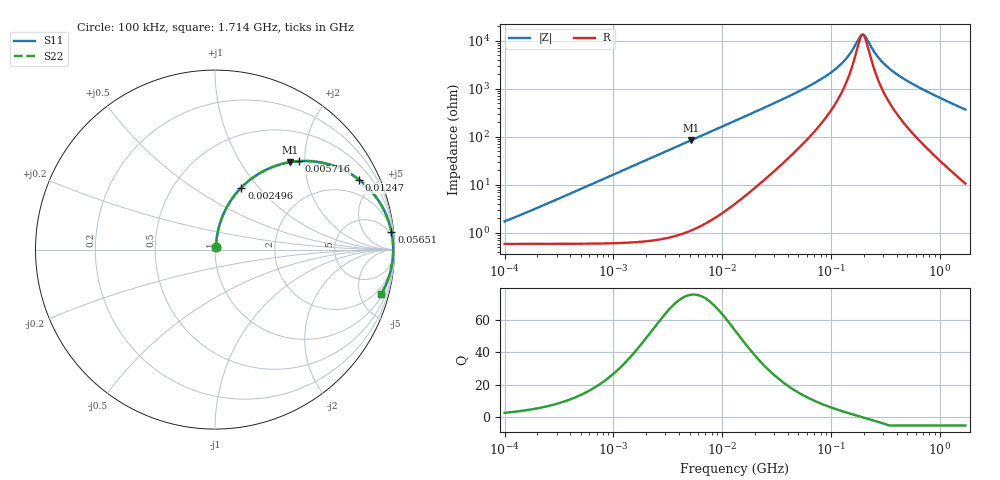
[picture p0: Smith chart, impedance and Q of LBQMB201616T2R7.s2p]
! LBQMB201616T2R7  S-PARAMETER MODEL  ( General Type )
! Model Generated by TAIYO YUDEN Corporation (http://www.ty-top.com)
! Version 1.0
! TAIYO YUDEN Control No. 191025NI43SB-FBB
! Copyright(c) 2019 TAIYO YUDEN CO.,LTD. All Rights Reserved.
! Product Description (link to TY-COMPAS)
! https://ds.yuden.co.jp/TYCOMPAS/or/detail?pn=LBQMB201616T2R7J&u=M
! Products Name : Inductors
! Characteristics :
!  Inductance : 2.7 uH , SRF(min) : 55 MHz , DC Resistance(max) : 0.767 Ohm , Rated Current : 310 mA
!  Case Size : 2.0 x 1.6 / 0.079 x 0.063 [mm/inch] , Thickness : 1.6 / 0.063 [mm/inch]
!  (Conditions: Temperature = 25 degC , DC Bias Current/Voltage = 0A / 0V)
! External Node Assignments :
!  1  o---GGG---o  2
! GND o---------o GND
! Frequency Range : 0.1MHz  -  1713.942084MHz  [ 402 STEP ]
# MHz S RI R 50
! Freq[MHz].  S11 Real  S11 Imag  S21 Real  S21 Imag  S12 Real  S12 Imag  S22 Real  S22 Imag
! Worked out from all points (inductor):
!   401 points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, 100 kHz to 1.714 GHz, reference 50 ohm
!   read as one part in series: L = 2.6 uH near 110.2 kHz
!   highest Q = 75.5 at 5.185 MHz (marker M1), where L = 2.61 uH
!   self-resonance near 191.1 MHz
!   S11 on the Smith chart (normalised r, x): 100 kHz: 1.01, +0.03; 2.496 MHz: 1.01, +0.82; 5.716 MHz: 1.02, +1.87; 12.47 MHz: 1.07, +4.09; 56.51 MHz: 3, +20; 1.714 GHz: 1.21, -7.37
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0.1  0.00613 0.0162  0.9939 -0.0162  0.9939 -0.0162  0.00613 0.0162
0.511911  0.0128 0.0822  0.9872 -0.0822  0.9872 -0.0822  0.0128 0.0822
1.324369  0.0502 0.2045  0.9498 -0.2045  0.9498 -0.2045  0.0502 0.2045
2.495851  0.1473 0.3457  0.8527 -0.3457  0.8527 -0.3457  0.1473 0.3457
2.620527  0.1595 0.3578  0.8405 -0.3578  0.8405 -0.3578  0.1595 0.3578
5.185235  0.4198 0.487  0.5802 -0.487  0.5802 -0.487  0.4198 0.487
5.716213  0.4673 0.4924  0.5327 -0.4924  0.5327 -0.4924  0.4673 0.4924
12.4689  0.8031 0.3887  0.1969 -0.3887  0.1969 -0.3887  0.8031 0.3887
13.41476  0.8247 0.3708  0.1753 -0.3708  0.1753 -0.3708  0.8247 0.3708
24.07813  0.9348 0.2319  0.0652 -0.2319  0.0652 -0.2319  0.9348 0.2319
56.50638  0.9831 0.0967  0.0169 -0.0967  0.0169 -0.0967  0.9831 0.0967
67.01815  0.9863 0.0788  0.0137 -0.0788  0.0137 -0.0788  0.9863 0.0788
94.27191  0.9902 0.0489  0.00978 -0.0489  0.00978 -0.0489  0.9902 0.0489
123.2586  0.9918 0.0294  0.00823 -0.0294  0.00823 -0.0294  0.9918 0.0294
149.7949  0.9924 0.0165  0.00763 -0.0165  0.00763 -0.0165  0.9924 0.0165
182.0443  0.9926 0.00432  0.00737 -0.00432  0.00737 -0.00432  0.9926 0.00432
195.8538  0.9926 -0.000192  0.00735 0.000192  0.00735 0.000192  0.9926 -0.000192
210.7109  0.9926 -0.00471  0.00738 0.00471  0.00738 0.00471  0.9926 -0.00471
268.8666  0.9922 -0.0201  0.00776 0.0201  0.00776 0.0201  0.9922 -0.0201
343.0732  0.9913 -0.0366  0.00871 0.0366  0.00871 0.0366  0.9913 -0.0366
630.9741  0.9845 -0.0894  0.0155 0.0894  0.0155 0.0894  0.9845 -0.0894
1713.942  0.9252 -0.249  0.0748 0.249  0.0748 0.249  0.9252 -0.249
